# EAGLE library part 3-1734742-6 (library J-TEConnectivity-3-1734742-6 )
36 Position FFC, FPC Connector Contacts, Vertical, 1 Sided 0.020" (0.50mm) Surface Mount
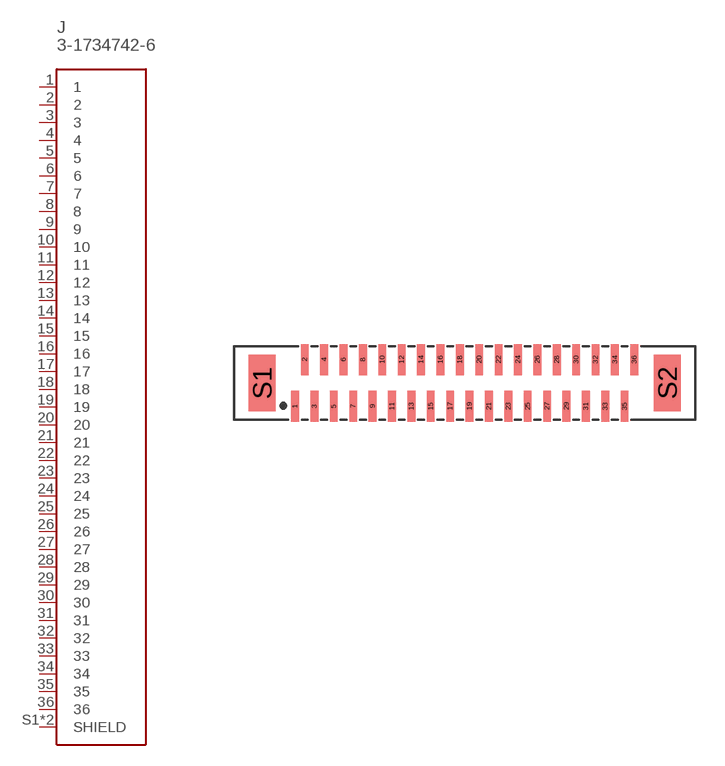
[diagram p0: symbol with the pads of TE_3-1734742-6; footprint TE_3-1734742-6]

Designator prefix J

## 3-1734742-6 (COMMENT: 4-1734742-0; DESCRIPTION: Conn FPC Connector SKT 36 POS 0.5mm Solder ST SMD T/R; DIGI-KEY_PART_NUMBER: A100242CT-ND; MF: TE Connectivity; MP: 4-1734742-0; PACKAGE: None)  [TE_3-1734742-6]
1  1  pas
2  2  pas
3  3  pas
4  4  pas
5  5  pas
6  6  pas
7  7  pas
8  8  pas
9  9  pas
10  10  pas
11  11  pas
12  12  pas
13  13  pas
14  14  pas
15  15  pas
16  16  pas
17  17  pas
18  18  pas
19  19  pas
20  20  pas
21  21  pas
22  22  pas
23  23  pas
24  24  pas
25  25  pas
26  26  pas
27  27  pas
28  28  pas
29  29  pas
30  30  pas
31  31  pas
32  32  pas
33  33  pas
34  34  pas
35  35  pas
36  36  pas
S1  SHIELD  pas
S2  SHIELD  pas

## Footprint TE_3-1734742-6 (pad centres in mm)
smd 0.4 x 1.6: 1 -9.75,-1.2; 2 -9.25,1.2; 3 -8.75,-1.2; 4 -8.25,1.2; 5 -7.75,-1.2; 6 -7.25,1.2; 7 -6.75,-1.2; 8 -6.25,1.2; 9 -5.75,-1.2; 10 -5.25,1.2; 11 -4.75,-1.2; 12 -4.25,1.2; 13 -3.75,-1.2; 14 -3.25,1.2; 15 -2.75,-1.2; 16 -2.25,1.2; 17 -1.75,-1.2; 18 -1.25,1.2; 19 -0.75,-1.2; 20 -0.25,1.2; 21 0.25,-1.2; 22 0.75,1.2; 23 1.25,-1.2; 24 1.75,1.2; 25 2.25,-1.2; 26 2.75,1.2; 27 3.25,-1.2; 28 3.75,1.2; 29 4.25,-1.2; 30 4.75,1.2; 31 5.25,-1.2; 32 5.75,1.2; 33 6.25,-1.2; 34 6.75,1.2; 35 7.25,-1.2; 36 7.75,1.2
smd 1.4 x 2.9: S1 -11.45,0; S2 9.45,0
